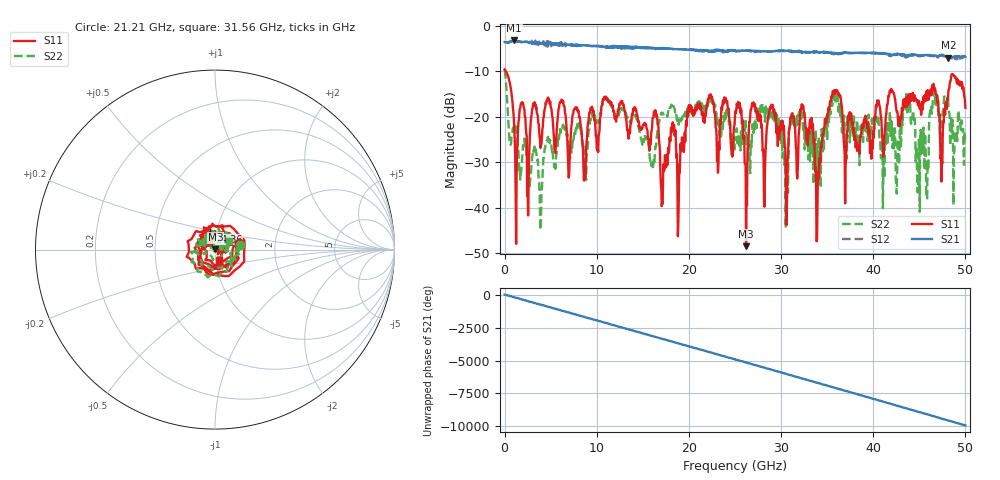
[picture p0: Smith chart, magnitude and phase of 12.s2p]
! 2/2/2024 4:23:22 PM
! D:\_XLC\ZPD9-2M1-50G-2425\12.S2P
! CHANNEL.1
! TR.MEASUREMENT
! CORRECTED.DATA
! RF.CORRECTION: FULL.TWO.PORT.CAL.PORT.1.2
! AVERAGING.OFF
! IF.BANDWIDTH: NO.IFBW
! SWEEPTYPE:  FREQ.SWEEP(Linear)
! Reference Plane Port Info
! PORT:  PORT1  PORT2
! DISTANCE:  0  m  0  m
! TIME:  0  s  0  s
! PHASE.OFFSET:  0 °  0 °
! LOSS:  0  dB  0  dB
! REF.LOSS:  0  dB  0  dB
! REF.FREQ:  0  Hz  0  Hz
! Power Info
! POWER:  0  dBm  0  dBm
! EFF.POWER:  0  dBm  0  dBm
! SOURCE.ATTEN:  0  dB  0  dB
! TEST.ATTEN:  0  dB  0  dB
# GHZ S RI R 50.0
! FREQ.GHZ  S11RE  S11IM  S21RE  S21IM  S12RE  S12IM  S22RE  S22IM
!; PortSelection: Port_12
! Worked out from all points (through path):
!   1001 points, 10 MHz to 50.01 GHz, reference 50 ohm
!   highest |S21| = -3.25 dB at 1.06 GHz (marker M1); lowest = -7.1 dB at 48.16 GHz (marker M2)
!   group delay of S21, straight-line fit = 550 ps
!   lowest |S11| = -48.5 dB at 26.21 GHz (marker M3), VSWR 1.01, Z = 50.3 + j0.272 ohm
!   |S11| at or under -10 dB: 140.9 MHz to end of sweep
!   |S22| runs from -45.0 to -9.7 dB; largest |S21 - S12| = 0.065
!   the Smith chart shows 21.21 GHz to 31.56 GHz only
!   S11 on the Smith chart (normalised r, x): 21.21 GHz: 1.31, +0.09; 24.36 GHz: 0.92, +0.19; 31.56 GHz: 1.04, -0.12
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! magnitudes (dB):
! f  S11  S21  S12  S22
! 10 MHz  -9.6  -3.6  -3.6  -9.7
! 1.06 GHz  -23.1  -3.2  -3.4  -21.9
! 3.91 GHz  -26.9  -3.8  -3.9  -45.0
! 8.36 GHz  -23.1  -4.3  -4.3  -23.7
! 16.71 GHz  -22.5  -4.9  -4.9  -21.3
! 18.91 GHz  -38.0  -5.1  -5.2  -21.8
! 21.21 GHz  -17.2  -5.6  -5.5  -17.1
! 24.36 GHz  -19.6  -5.6  -5.5  -21.8
! 25.01 GHz  -19.9  -5.5  -5.6  -24.6
! 26.21 GHz  -48.5  -5.4  -5.5  -22.7
! 26.96 GHz  -17.5  -5.6  -5.6  -22.5
! 30.56 GHz  -42.5  -5.5  -5.6  -33.8
! 31.56 GHz  -23.9  -5.7  -5.8  -20.7
! 33.36 GHz  -22.7  -5.9  -5.9  -26.7
! 33.96 GHz  -39.8  -5.8  -5.8  -29.7
! 35.71 GHz  -15.1  -6.1  -6.3  -15.7
! 37.01 GHz  -30.9  -5.8  -6.0  -24.3
! 41.71 GHz  -15.5  -6.2  -6.6  -23.1
! 46.61 GHz  -13.5  -6.5  -6.7  -14.4
! 47.41 GHz  -34.3  -6.4  -6.5  -21.2
! 48.16 GHz  -14.5  -7.1  -6.9  -17.1
! 50.01 GHz  -18.1  -6.9  -6.9  -23.9
